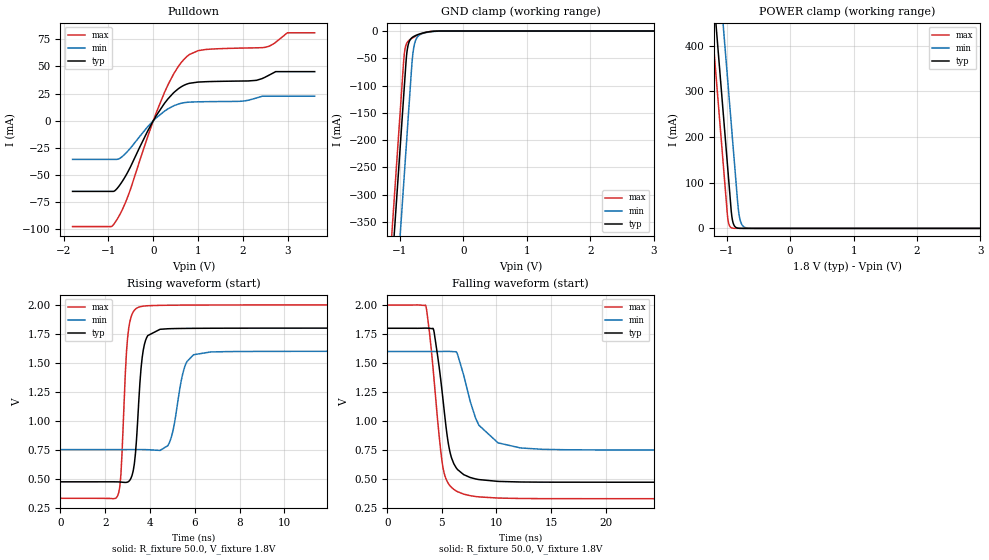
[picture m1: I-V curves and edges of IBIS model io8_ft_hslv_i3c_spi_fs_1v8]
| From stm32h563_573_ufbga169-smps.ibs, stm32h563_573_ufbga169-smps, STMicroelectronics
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[Model]   io8_ft_hslv_i3c_spi_fs_1v8
Model_type I/O_open_drain
Polarity   Non-Inverting
Enable   Active-Low
| CAP_THRESHOLD on pad IOFT is "UDTCAPC" :
| Rising=20.0% of vddiom   Falling=80.0% of vddiom
| C_comp min and max val. don't necessarily correlate with the min and max pvt
| but are the smallest and greatest pad capacitance found.
| var   typ   min   max
C_comp   3.75311pF  3.69067pF  3.87717pF
|C_comp_pulldown   3.75311pF  3.69067pF  3.87717pF
Vinl = 800.0mV
Vinh = 1.0V
Vmeas = 900.0mV   | Reference voltage for timing measurements
Cref  = 50.0pF   | Timing specification test load capacitance value
Rref  = 1.0MOhm   | Timing specification test load resistance value
Vref  = 990.0mV   | Timing specification test load voltage
[Model Spec]
| TIME_THRESHOLD on pin ZII2CV11 is "CMOS" :
| Rising=40.0% of vdd   Falling=60.0% of vdd
Vinl 703.80000mV 631.80000mV 784.80000mV
Vinh 1.06220V 937.20000mV 1.16620V
| variable   typ   min   max
[Temperature Range] 25.0 125.0 -40.0
| variable   typ   min   max
[Voltage Range] 1.8V 1.6V 2.0V
| variable   typ   min   max
[POWER Clamp Reference] 1.8V 1.6V 2.0V
| variable   typ   min   max
[GND Clamp Reference] 0V 0V 0V
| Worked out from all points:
|   slope of the pulldown table from 0 to 0.27 V, typ, clamps not added: 15.8 ohm
|   GND clamp passes 1 mA (typ) near -0.52 V on its own axis
|   POWER clamp passes 1 mA (typ) near -0.84 V on its own axis
|   rising waveform, R_fixture 50.0, V_fixture 1.8V: 20-80 % time 286ps typ, 462ps min, 244ps max; typ from 0.474 V to 1.8 V
|   falling waveform, R_fixture 50.0, V_fixture 1.8V: 20-80 % time 1.08ns typ, 2ns min, 1.02ns max; typ from 1.8 V to 0.474 V
[POWER Clamp]
-1.8V     1.518A     1.709A     1.407A
-1.23V    548.8mA    740.2mA    437.5mA
-1.16V    429.8mA    621.2mA    318.5mA
-1.05V    242.8mA    434.2mA    131.5mA
-980mV    123.8mA    315.2mA    17.95mA
-930mV    38.81mA    230.2mA    1.49mA
-910mV    17.82mA    196.2mA    550.8uA
-890mV    8.18mA     162.2mA    203.5uA
-810mV    363.5uA    33.6mA     3.797uA
-770mV    76.62uA    10.47mA    518.8nA
-710mV    7.416uA    1.822mA    26.34nA
3.6V      0A         0A         0A
[GND Clamp]
-1.8V     -1.579A    -1.74A     -1.515A
-1.24V    -627.3mA   -788.3mA   -562.7mA
-1.05V    -304.3mA   -465.3mA   -239.7mA
-940mV    -117.3mA   -278.3mA   -52.69mA
-930mV    -100.3mA   -261.3mA   -40.52mA
-900mV    -50.11mA   -210.3mA   -24.23mA
-880mV    -30.95mA   -176.3mA   -20.02mA
-810mV    -12.18mA   -57.97mA   -13.23mA
-780mV    -9.807mA   -29.1mA    -11.19mA
-690mV    -5.41mA    -7.142mA   -6.184mA
-420mV    -170.4uA   -446.1uA   -81.94uA
3.6V      5.755nA    953.4nA    228.2pA
| variable   typ   min   max
[Pullup Reference] 1.8V 1.6V 2.0V
| variable   typ   min   max
[Pulldown Reference] 0V 0V 0V
[Pulldown]
-1.8V     -65.02mA   -35.56mA   -97.42mA
-940mV    -65.02mA   -35.56mA   -97.42mA
-850mV    -64.17mA   -35.56mA   -93.49mA
-570mV    -47.32mA   -28.01mA   -70.04mA
-120mV    -9.088mA   -5.279mA   -14.07mA
250mV     16.04mA    8.832mA    26.05mA
550mV     29.17mA    15.25mA    49.41mA
780mV     34.17mA    17.07mA    60.14mA
1.18V     35.97mA    17.56mA    65.65mA
2.49V     40mA       22.62mA    67.56mA
2.99V     45.21mA    22.62mA    80.94mA
3.6V      45.21mA    22.62mA    80.94mA
[Ramp]
dV/dt_r 795.76527mV/284.05972ps 508.9486mV/461.08976ps 1.00097V/239.6563ps
dV/dt_f 795.78722mV/1.07778ns 508.98182mV/1.78967ns 1.00099V/1.02319ns
R_load = 50.0
| Removed startup time: 0s 0s 0s  .
| Removed end time: 36.4ns.
[Rising Waveform]
R_fixture   = 50.0
V_fixture   = 1.8V
V_fixture_min = 1.6V
V_fixture_max = 2.0V
0s        473.7mV    751.7mV    331.7mV
2.55ns    473.3mV    751.8mV    350.7mV
2.7ns     471.7mV    751.8mV    533mV
3.05ns    477.1mV    752mV      1.799V
3.3ns     626.3mV    752mV      1.954V
3.6ns     1.451V     752mV      1.986V
4.8ns     1.794V     786.2mV    1.997V
5.6ns     1.797V     1.491V     1.998V
6.7ns     1.799V     1.594V     1.999V
36.4ns    1.8V       1.6V       2V
| Removed startup time: 0s 0s 0s  .
| Removed end time: 99.4ns.
[Falling Waveform]
R_fixture   = 50.0
V_fixture   = 1.8V
V_fixture_min = 1.6V
V_fixture_max = 2.0V
0s        1.8V       1.6V       2V
3.5ns     1.801V     1.6V       1.999V
4.25ns    1.786V     1.6V       1.397V
5.2ns     1.104V     1.601V     556.9mV
5.9ns     680.1mV    1.6V       427.7mV
6.4ns     587.3mV    1.584V     393.8mV
7.6ns     514.2mV    1.169V     357.7mV
10.15ns   480.7mV    812.8mV    337.1mV
14.2ns    474.2mV    757.2mV    332.3mV
99.4ns    473.7mV    751.7mV    331.7mV
